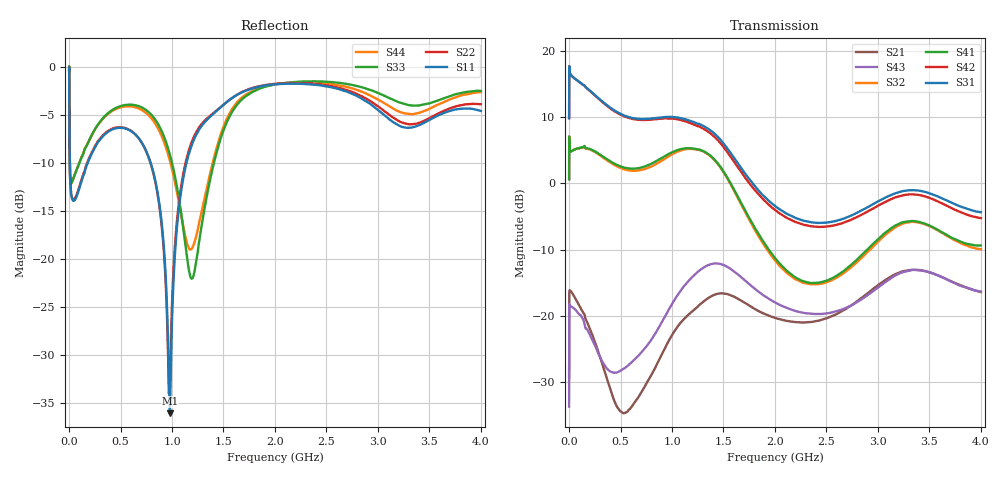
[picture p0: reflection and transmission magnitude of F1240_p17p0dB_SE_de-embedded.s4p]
! Integrated Device Technology
! Corporate Headquarters
! 6024 Silver Creek Valley Road
! San Jose, CA 95138  USA
! Phone:  1-408-284-8200
! Toll Free:  1-800-223-1366
! Webpage:  http://www.idt.com/
! Timing and RF Division
! 515 Groton Road, Suite 102
! Westford, MA 01886-6024
! Device:  F1240
! Description: Dual Intermediate Frequency Digital Variable Gain Amplifier
! Frequency:  10.0 -  500.00 MHz
! Package:  5x5 mm QFN Plastic Package: 32 pin
! Ports:  8 RF, 20 DC
!  Pin  1  = GA3 / Data  Pin 17  = RF OUT_B+
!  Pin  2  = GA4 / CLK  Pin 18  = RF OUT_B-
!  Pin  3  = GA5  Pin 19  = STBY_B
!  Pin  4  = VMODE  Pin 20  = Ground
!  Pin  5  = No Connect  Pin 21  = Ground
!  Pin  6  = GB5  Pin 22  = STB_A
!  Pin  7  = GB4  Pin 23  = RF OUT_A-  = Port 4
!  Pin  8  = GB3  Pin 24  = RF OUT_A+  = Port 3
!  Pin  9  = GB2  Pin 25  = GA0
!  Pin 10  = GB1  Pin 26  = ISET_A
!  Pin 11  = RF IN_B+  Pin 27  = VCC
!  Pin 12  = RF IN_B-  Pin 28  = Ground
!  Pin 13  = Ground  Pin 29  = RF IN_A-  = Port 2
!  Pin 14  = VCC  Pin 30  = RF IN_A+  = Port 1
!  Pin 15  = ISET_B  Pin 31  = GA1
!  Pin 16  = GB0  Pin 32  = GA2 / CSb
! Gain  = +19.5 dB
! State  = 1
! Voltage  = +5.00 V
! Current  = 85.292 mA (one channel only)
! Temperture  =  +25 C
! Test Date  =  2017-10-18
! Board  =  EB4031
! Data:  The device was measured on a custom evaluation board which has
!  individual transmission lines to the RF pins.  Data was collected
!  using a calibrated network analyzer.  The evaluation board was
!  de-embedded using Automatic Fixture Removal.
!  The reference plane is the edge of the package pin.
!  Only Channel A was measured.
!  This data is in single-ended operation.  If your needs are balanced
!  or differential S-parameters then this file needs to be used a
!  linear simulator.
! File Date:  2017-11-10  MJV
! Note:
!  Integrated Device Technology supplies this data as a sample of measured
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# Hz S dB R 100
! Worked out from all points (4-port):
!   410 points, 500 kHz to 4 GHz, reference 100 ohm
!   strongest paths, dB at 500 kHz, 930 MHz, 1.96 GHz, 2.98 GHz, 4 GHz:
!     S31: 9.8, 10.0, -2.9, -2.9, -4.4
!     S42: 9.8, 9.8, -3.5, -3.6, -5.2
!     S41: 0.6, 4.1, -10.4, -8.7, -9.4
!     S32: 0.6, 3.7, -10.8, -9.1, -9.9
!     S43: -33.7, -20.1, -17.6, -16.0, -16.3
!     S21: -29.3, -24.9, -20.1, -15.6, -16.4
!   lowest |S11| = -36.0 dB at 980 MHz (marker M1), VSWR 1.03, Z = 103 + j0.475 ohm
!   |S11| at or under -10 dB: 7.549 MHz to 181.4 MHz (173.9 MHz wide, 184 % of centre); 792.6 MHz to 1.14 GHz (347.5 MHz wide, 36 % of centre)
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500000  -0.32 -6.4  -29.22 13.2  -27.48 73.1  -62.50 65.2
        -29.30 13.0  -0.32 -6.3  -61.92 64.9  -27.50 74.3
        9.83 -105.4  0.62 72.4  -0.43 0.9  -33.69 -164.8
        0.61 73.5  9.81 -104.3  -33.68 -164.8  -0.44 3.2
3000000  -4.99 -49.7  -16.40 18.4  -20.34 11.3  -40.02 53.0
         -16.41 18.4  -4.96 -49.8  -39.99 52.8  -20.35 11.5
         17.40 -169.3  5.73 -0.4  -4.61 -44.8  -18.23 34.6
         5.72 -0.3  17.39 -169.1  -18.20 34.5  -4.67 -44.5
2.1e8  -9.27 -112.4  -22.17 -110.8  -23.31 -53.3  -33.42 8.8
       -22.22 -109.5  -9.13 -114.1  -33.45 8.9  -23.33 -53.2
       13.89 105.9  5.04 -59.8  -7.33 -80.8  -22.52 -122.5
       5.13 -59.7  13.83 105.1  -23.10 -121.2  -7.34 -80.2
5.6e8  -6.47 -173.8  -33.63 74.5  -24.96 -108.9  -27.56 -61.5
       -34.52 68.5  -6.43 -175.1  -27.73 -60.2  -25.13 -109.2
       10.08 20.1  2.01 -140.8  -3.96 -152.4  -27.60 75.1
       2.29 -141.8  9.96 19.0  -27.64 53.8  -4.12 -152.0
9.8e8  -36.03 8.4  -21.63 -40.9  -22.02 165.0  -22.82 -160.8
       -23.42 -44.6  -32.78 -13.1  -23.18 -156.3  -22.48 164.4
       10.02 -81.4  4.18 128.8  -9.17 145.1  -18.36 -21.9
       4.52 123.9  9.79 -83.3  -18.74 -42.9  -9.81 149.8
1.51e9  -3.87 -141.9  -16.55 162.1  -28.50 40.8  -24.66 68.5
        -16.63 167.0  -3.86 -142.7  -24.63 74.4  -30.04 37.6
        5.82 120.2  1.44 -51.8  -6.33 -119.6  -12.26 158.1
        1.55 -56.8  5.28 118.7  -12.38 151.0  -5.96 -123.5
4e9  -4.61 -157.8  -16.43 56.8  -21.89 -37.0  -19.38 -48.2
     -16.41 56.2  -3.90 -151.2  -21.93 -29.7  -25.64 -20.0
     -4.36 2.3  -9.94 -132.2  -2.52 -135.9  -14.90 90.5
     -9.37 -142.4  -5.25 11.4  -16.33 63.8  -2.63 -140.9
